PROGRAM p10_blokadaSmeri
VAR
	blokadaS0: TOF;
	blokadaS1: TOF;
	S0: BOOL;	
	S1: BOOL;
	L0: BOOL;
	L1: BOOL;
END_VAR

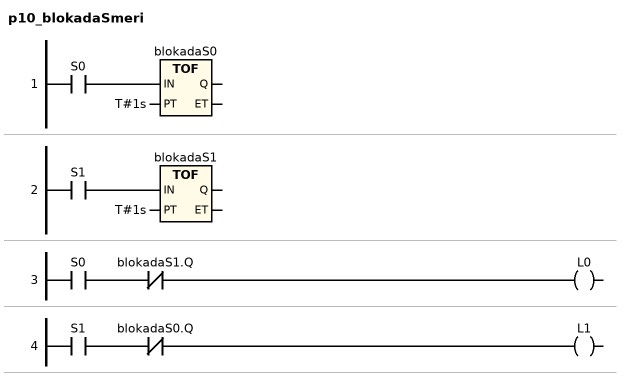
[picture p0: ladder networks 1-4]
// NETWORK 1
blokadaS0(IN := S0, PT := T#1s); // TOF

// NETWORK 2
blokadaS1(IN := S1, PT := T#1s); // TOF

// NETWORK 3
L0 := S0 AND NOT blokadaS1.Q;

// NETWORK 4
L1 := S1 AND NOT blokadaS0.Q;

END_PROGRAM
